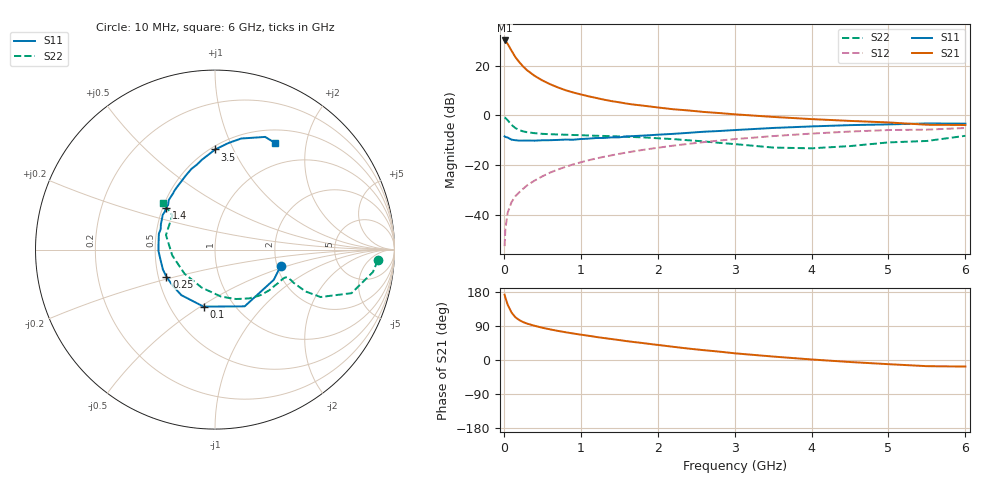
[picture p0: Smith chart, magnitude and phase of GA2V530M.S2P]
! Infineon Technologies  Discrete & RF Semiconductors
! BF775
! Si NPN RF Bipolar Junction Transistor in SOT23
! VCE = 2.5 V  IC = 30 mA
! Common Emitter S-Parameters:  May  1996
# GHz  S  MA  R  50
!  f  S11  S21  S12  S22
! GHz  MAG  ANG  MAG  ANG  MAG  ANG  MAG  ANG
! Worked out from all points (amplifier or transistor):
!   36 points, 10 MHz to 6 GHz, reference 50 ohm
!   highest |S21| = 30.2 dB at 10 MHz (marker M1)
!   |S21| within 3 dB of that: start of sweep to 79.17 MHz
!   unconditionally stable (mu >= 1): 186.7 MHz to end of sweep
!   at 250 MHz: K = 1.11, MAG = 22.7 dB, |S12| = -29.6 dB
!   at 1.4 GHz: K = 1.25, MAG = 7.9 dB, |S12| = -16.1 dB
!   at 6 GHz: K = 1.04, MAG = -0.7 dB, |S12| = -5.1 dB
!   S11 on the Smith chart (normalised r, x): 10 MHz: 2.10, -0.44; 100 MHz: 0.73, -0.52; 250 MHz: 0.55, -0.18; 1.4 GHz: 0.52, +0.28; 3.5 GHz: 0.53, +0.85; 6 GHz: 0.67, +1.49
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0.01  0.3777 -13.7  32.49 172.3  0.0023 86.8  0.9088 -3.8
0.02  0.3682 -27.2  31.72 164.7  0.0051 75.9  0.8888 -8.1
0.05  0.3567 -62.4  27.63 145.8  0.0109 72.6  0.7984 -17.7
0.1  0.324 -101.3  20.18 125.3  0.0178 66.8  0.6446 -24.2
0.15  0.3156 -126.5  14.99 112.8  0.0235 66.1  0.5548 -24.8
0.2  0.3097 -140.0  11.9 105.5  0.028 67.3  0.5061 -23.7
0.25  0.3099 -150.9  9.73 100.1  0.033 68.2  0.4765 -22.9
0.3  0.3108 -159.1  8.198 96.2  0.0385 70.5  0.4587 -22.0
0.4  0.3092 -170.4  6.276 90.3  0.0485 71.2  0.4377 -21.2
0.5  0.3149 -178.6  5.081 85.1  0.0589 72.6  0.4246 -21.3
0.6  0.3159 175.1  4.267 80.9  0.07 72.5  0.4175 -22.1
0.7  0.32 168.4  3.681 76.9  0.0807 72.5  0.4123 -23.1
0.8  0.3249 164.2  3.227 73.3  0.0915 71.7  0.4078 -24.5
1.1  0.3399 150.7  2.429 64.0  0.1243 69.7  0.3936 -29.5
1.4  0.3601 139.4  1.941 55.3  0.1564 67.1  0.3809 -35.2
1.7  0.3831 130.1  1.645 47.2  0.1896 63.8  0.3652 -41.9
2.2  0.424 116.2  1.331 34.9  0.2449 57.9  0.3326 -54.7
3  0.5057 98.3  1.052 17.7  0.3322 47.1  0.2635 -82.8
3.5  0.5578 89.9  0.932 9.1  0.3824 39.8  0.2244 -109.2
4.5  0.6361 76.7  0.774 -5.3  0.472 24.8  0.2404 -172.3
5.5  0.6873 66.0  0.648 -16.3  0.5159 9.1  0.3049 141.0
6  0.6819 60.8  0.639 -17.3  0.5568 4.7  0.3874 138.2
